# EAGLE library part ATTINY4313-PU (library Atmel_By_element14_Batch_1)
8-bit Microcontroller
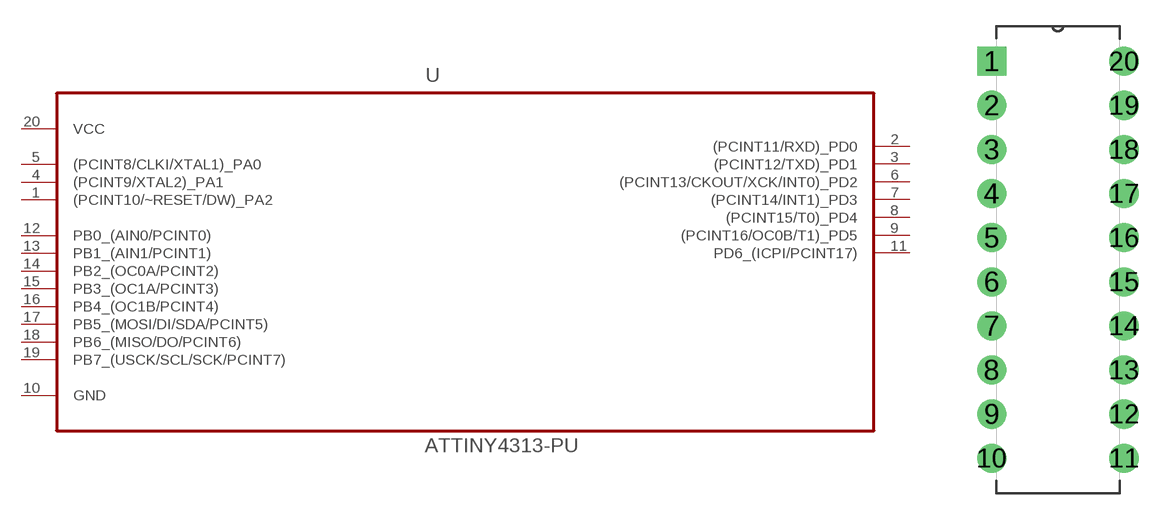
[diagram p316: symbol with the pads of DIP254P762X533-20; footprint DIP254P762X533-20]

Designator prefix U

## ATTINY4313-PU (DESCRIPTION: 8-bit Microcontroller; MPN: ATTINY4313-PU; OC_FARNELL: 1841620; OC_NEWARK: 12T1339; PACKAGE: DIP-20; SUPPLIER: Atmel)  [DIP254P762X533-20]
1  (PCINT10/~RESET/DW)_PA2
2  (PCINT11/RXD)_PD0
3  (PCINT12/TXD)_PD1
4  (PCINT9/XTAL2)_PA1
5  (PCINT8/CLKI/XTAL1)_PA0
6  (PCINT13/CKOUT/XCK/INT0)_PD2
7  (PCINT14/INT1)_PD3
8  (PCINT15/T0)_PD4
9  (PCINT16/OC0B/T1)_PD5
10  GND  pas
11  PD6_(ICPI/PCINT17)
12  PB0_(AIN0/PCINT0)
13  PB1_(AIN1/PCINT1)
14  PB2_(OC0A/PCINT2)
15  PB3_(OC1A/PCINT3)  pwr
16  PB4_(OC1B/PCINT4)  pas
17  PB5_(MOSI/DI/SDA/PCINT5)
18  PB6_(MISO/DO/PCINT6)
19  PB7_(USCK/SCL/SCK/PCINT7)
20  VCC  pwr

## Footprint DIP254P762X533-20 (pad centres in mm)
drill 1.118 square: 1 -7.62,22.86
drill 1.118: 2 -7.62,20.32; 3 -7.62,17.78; 4 -7.62,15.24; 5 -7.62,12.7; 6 -7.62,10.16; 7 -7.62,7.62; 8 -7.62,5.08; 9 -7.62,2.54; 10 -7.62,0; 11 0,0; 12 0,2.54; 13 0,5.08; 14 0,7.62; 15 0,10.16; 16 0,12.7; 17 0,15.24; 18 0,17.78; 19 0,20.32; 20 0,22.86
